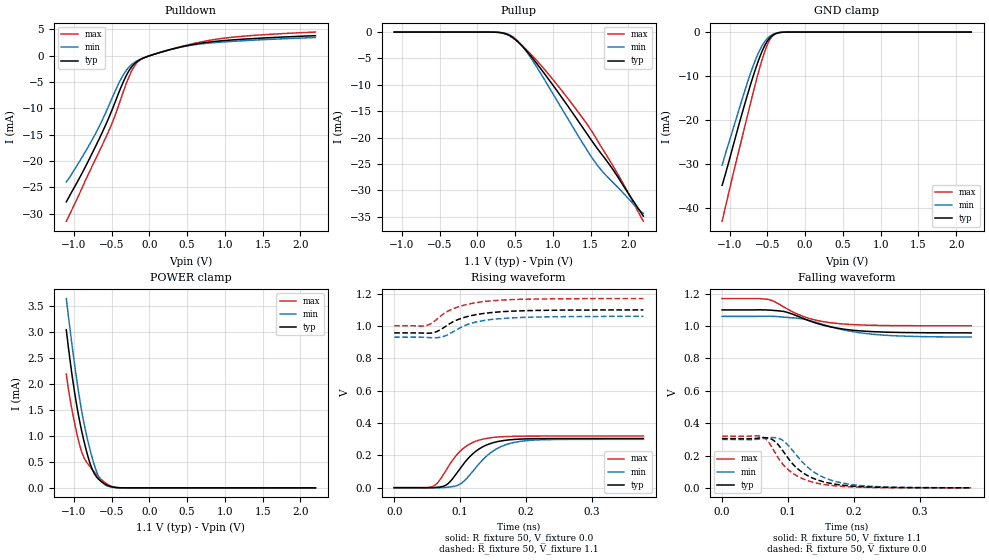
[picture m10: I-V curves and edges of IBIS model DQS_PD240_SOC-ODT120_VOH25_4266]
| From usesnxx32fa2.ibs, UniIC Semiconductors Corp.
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| DQS_PD240_SOC-ODT120_VOH25_4266
| (240 Ohm Pulldown, 120 Ohm System ODT Setting, VOH=VDDQ/2.5, 3200-4266Mbps)
[Model]   DQS_PD240_SOC-ODT120_VOH25_4266
Model_type   I/O
Vinl = 160.000mV
Vinh = 280.000mV
Vmeas = 220.000mV
Vref = 0.0mV
Cref = 0.0pF
Rref = 120.000Ohm
|   typ   min   max
|C_comp   0.849pF   0.799pF   0.899pF
C_comp_pullup   0.4245pF   0.3995pF   0.4495pF
C_comp_pulldown   0.4245pF   0.3995pF   0.4495pF
| Note: C_comp changes when the ODT circuit is enabled.
[Model Spec]
| Input threshold voltage corners
Vinl   0.1600V   0.1520V   0.1740V
Vinh   0.2800V   0.2720V   0.2940V
| Measurement voltage corners
Vmeas   0.2200V   0.2120V   0.2340V
| Timing spec test load voltage corners
Vref   0.0000V   0.0000V   0.0000V
| Dynamic Overshoot Parameters from LPDDR4 Specification
D_overshoot_ampl_h   0.30   NA   NA
D_overshoot_ampl_l   0.30   NA   NA
D_overshoot_area_h   0.1n   NA   NA
D_overshoot_area_l   0.1n   NA   NA
[Voltage Range]   1.1000V   1.0600V   1.1700V
[Pullup Reference]   1.1000V   1.0600V   1.1700V
| Junction Temperature (Ambient temp is 35C typ 95C min -40C max)
[Temperature Range]   50.0   110.0   -40.0
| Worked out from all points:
|   slope of the pulldown table from 0 to 0.165 V, typ, clamps not added: 223 ohm
|   slope of the pullup table from 0 to 0.165 V, typ, clamps not added: 26.3 kohm
|   GND clamp passes 1 mA (typ) near -0.45 V on its own axis
|   POWER clamp passes 1 mA (typ) near -0.88 V on its own axis
|   rising waveform, R_fixture 50, V_fixture 0.0: 20-80 % time 40.6ps typ, 44.3ps min, 36.9ps max; typ from 0.001 V to 0.305 V
|   falling waveform, R_fixture 50, V_fixture 1.1: 20-80 % time 67.7ps typ, 78.6ps min, 57.5ps max; typ from 1.1 V to 0.958 V
|   rising waveform, R_fixture 50, V_fixture 1.1: 20-80 % time 51.9ps typ, 50.2ps min, 50.5ps max; typ from 0.958 V to 1.1 V
|   falling waveform, R_fixture 50, V_fixture 0.0: 20-80 % time 47.4ps typ, 51.5ps min, 43.3ps max; typ from 0.305 V to 0.001 V
[Pulldown]
|   Voltage   I(typ)   I(min)   I(max)
-1.1V     -27.78mA   -23.99mA   -31.46mA
-928.4mV  -23.32mA   -20.17mA   -26.31mA
-720.5mV  -17.47mA   -15mA      -19.88mA
-506mV    -10.72mA   -8.467mA   -13.25mA
-344.3mV  -4.949mA   -3.634mA   -6.825mA
-232.1mV  -2.078mA   -1.645mA   -2.848mA
-133.1mV  -832.5uA   -755.8uA   -927.9uA
0V        -19.79uA   -16.35uA   -14.41uA
375.1mV   1.526mA    1.497mA    1.571mA
863.5mV   2.71mA     2.491mA    3.084mA
1.391V    3.275mA    2.965mA    3.873mA
2.2V      3.814mA    3.471mA    4.502mA
[GND Clamp]
|   Voltage   I(typ)   I(min)   I(max)
-1.1V     -34.75mA   -30.2mA    -42.92mA
-1.027V   -30.44mA   -26.03mA   -37.57mA
-935mV    -24.61mA   -20.88mA   -30.86mA
-789.8mV  -15.73mA   -12.78mA   -20.73mA
-667.7mV  -8.911mA   -6.72mA    -12.3mA
-591.8mV  -5.257mA   -3.788mA   -7.499mA
-525.8mV  -2.767mA   -1.975mA   -3.966mA
-469.7mV  -1.356mA   -985.5uA   -1.789mA
-413.6mV  -564uA     -417.2uA   -620.9uA
-357.5mV  -191.5uA   -144.5uA   -173.6uA
-255.2mV  -14.7uA    -12.98uA   -8.827uA
2.2V      0A         0A         0A
[Pullup]
|   Voltage   I(typ)   I(min)   I(max)
-1.1V     2.737uA    4.954uA    907.4nA
262.9mV   -43.17uA   -41.94uA   -44.28uA
391.6mV   -403.5uA   -335.7uA   -480uA
497.2mV   -1.327mA   -1.186mA   -1.397mA
609.4mV   -2.879mA   -2.883mA   -2.763mA
748mV     -5.234mA   -5.722mA   -4.774mA
1.042V    -10.85mA   -12.64mA   -9.701mA
1.425V    -18.69mA   -21.71mA   -16.87mA
1.642V    -23.05mA   -26.16mA   -21.76mA
1.887V    -28.02mA   -29.79mA   -27.54mA
2.101V    -32.76mA   -33.11mA   -33.27mA
2.2V      -34.89mA   -34.37mA   -35.86mA
[POWER Clamp]
|   Voltage   I(typ)   I(min)   I(max)
-1.1V     3.033mA    3.633mA    2.184mA
-1.054V   2.491mA    3.082mA    1.736mA
-977.9mV  1.723mA    2.241mA    1.16mA
-911.9mV  1.2mA      1.61mA     764.7uA
-852.5mV  818.3uA    1.148mA    543.6uA
-779.9mV  447.9uA    701.4uA    396.3uA
-710.6mV  232.3uA    359.1uA    273.1uA
-654.5mV  142.6uA    170.5uA    185.9uA
-591.8mV  77.91uA    64.81uA    105.5uA
-492.8mV  18.88uA    11.57uA    24.03uA
-383.9mV  1.75uA     1.212uA    1.463uA
2.2V      0A         0A         0A
[Ramp]
|   typ   min   max
| 20% - 80%
dV/dt_r   182.39m/40.62p   179.46m/44.35p   191.72m/36.95p
dV/dt_f   85.15m/67.67p   76.64m/78.17p   100.79m/57.60p
| 25% - 75%
|dV/dt_r   151.99m/32.34p   149.55m/35.31p   159.76m/29.40p
|dV/dt_f   70.96m/53.84p   63.87m/62.06p   83.99m/45.83p
R_load = 50
[Rising Waveform]
R_fixture = 50
V_fixture = 0.0
|   Time   V(typ)   V(min)   V(max)
0s        784.6uV    650.2uV    572.4uV
57ps      544uV      -48.6uV    6.197mV
66ps      3.25mV     -232.8uV   31.87mV
77ps      13.23mV    2.004mV    97.6mV
104ps     141.6mV    34.51mV    240.9mV
121ps     216.5mV    111.2mV    283.4mV
138ps     260.8mV    188.2mV    304mV
163ps     290.5mV    256.6mV    315.6mV
195ps     301.8mV    289mV      319.3mV
378ps     304.8mV    299.7mV    320.1mV
[Falling Waveform]
R_fixture   = 50
V_fixture   = 1.1
V_fixture_min = 1.06
V_fixture_max = 1.17
|   Time   V(typ)   V(min)   V(max)
0s        1.1V       1.06V      1.17V
70ps      1.099V     1.061V     1.165V
77ps      1.097V     1.06V      1.156V
93ps      1.091V     1.056V     1.12V
124ps     1.046V     1.043V     1.058V
146ps     1.014V     1.019V     1.033V
170ps     990.7mV    990.6mV    1.018V
204ps     972.4mV    962mV      1.008V
246ps     962.9mV    943.9mV    1.004V
378ps     958.1mV    932.3mV    1.002V
[Rising Waveform]
R_fixture   = 50
V_fixture   = 1.1
V_fixture_min = 1.06
V_fixture_max = 1.17
|   Time   V(typ)   V(min)   V(max)
0s        957.9mV    931.6mV    1.002V
47ps      955.8mV    930.2mV    1.002V
57ps      957.6mV    928.1mV    1.018V
70ps      977.3mV    931mV      1.061V
88ps      1.024V     961.7mV    1.105V
103ps     1.05V      996.1mV    1.126V
117ps     1.065V     1.018V     1.14V
138ps     1.079V     1.036V     1.153V
210ps     1.096V     1.056V     1.167V
378ps     1.1V       1.06V      1.17V
[Falling Waveform]
R_fixture = 50
V_fixture = 0.0
|   Time   V(typ)   V(min)   V(max)
0s        304.9mV    299.8mV    320.2mV
61ps      310.2mV    304.1mV    315.8mV
71ps      307.4mV    309.8mV    280.3mV
86ps      262.5mV    306.3mV    179.1mV
98ps      195.1mV    273.2mV    121.2mV
115ps     117mV      191.2mV    71.22mV
146ps     47.48mV    81.59mV    27.47mV
174ps     21.53mV    37.98mV    11.89mV
213ps     7.608mV    13.66mV    3.994mV
378ps     933.1uV    922.8uV    632.4uV
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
